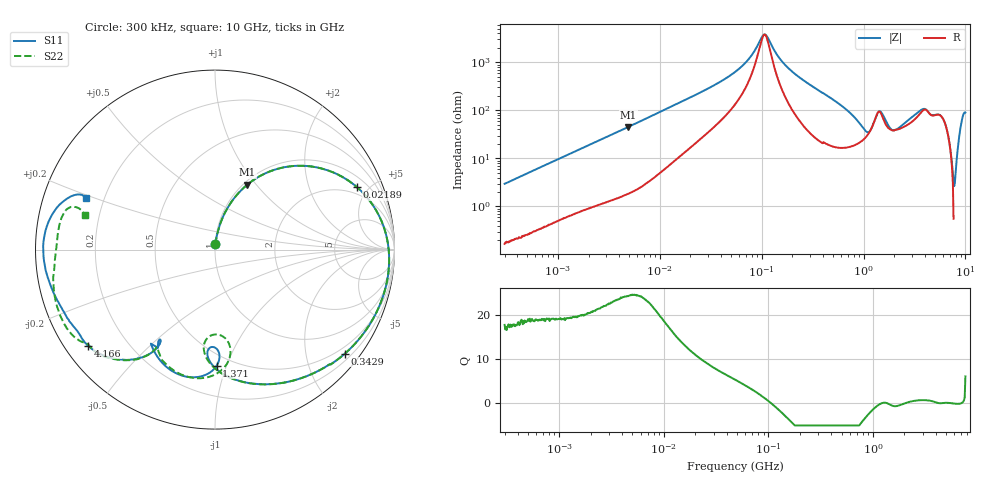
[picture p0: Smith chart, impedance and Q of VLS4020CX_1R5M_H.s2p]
! S-Parameter Data Generated by TDK Corporation
! Copyright(C) 2024 TDK Corporation.
! All Rights Reserved.
! TDK P/N: VLS4020CX-1R5M-H (SMD / SMT Inductor (Coil))
! Property: L=1.5uH at 1MHz
! Size(LxWxT): 4x4x2mm
! Model Type: s2p (Touchstone File Format Version 1.0)
! Frequency: DC=Yes Start=0.3MHz Stop=10000MHz 802points Log-sweep
! Model Generated on May 28, 2024
! Terms and conditions regarding TDK Simulation Models:
! 1)This simulation model is being provided solely for informational
!  purposes. Please refer to the specifications of the products in
!  terms of detailed characteristics of such products.
! 2)In no event shall TDK Corporation of any of its subsidiaries be
!  liable for any loss or damage arising, directly or indirectly,
!  from any information contained in this simulation model, including,
!  but not limited to loss or damages arising from any inaccuracies,
!  omissions or errors in connection with such information.
! 3)Any and all copyrights on this simulation model are owned by
!  TDK Corporation.  Duplication or redistribution of this simulation
!  model without prior written permission from TDK Corporation
!  is prohibited.
! 4)This simulation model is subject to any modification or change
!  without any prior notice.
! 5)Neither TDK Corporation nor any of its subsidiaries shall make any
!  warranty, express or implied, including but not limited to the
!  correctness, implied warranties of merchantability and fitness for
!  a particular purpose with respect to this simulation models.
! 6)The use of this simulation model shall be deemed to have consented
!  to the terms and conditions hereof.
! Port Assignments:
!  1 ---@@@--- 2
! Applicable Conditions:
!  Temperature = 25 degC
!  DC Bias Current = 0 A
!  Small Signal Operation
# Hz S MA R 50
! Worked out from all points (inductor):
!   801 points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, 300 kHz to 10 GHz, reference 50 ohm
!   read as one part in series: L = 1.56 uH near 318.3 kHz
!   highest Q = 24.6 at 4.921 MHz (marker M1), where L = 1.47 uH
!   self-resonance near 106.7 MHz
!   S11 on the Smith chart (normalised r, x): 300 kHz: 1.00, +0.06; 21.89 MHz: 1.54, +4.25; 342.9 MHz: 0.34, -2.81; 1.371 GHz: 0.42, -0.92; 4.166 GHz: 0.07, -0.33; 10 GHz: 0.13, +0.19
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300000  0.02934 85.0  0.998 -1.7  0.9978 -1.7  0.02926 85.1
1713600  0.1574 78.0  0.9796 -9.1  0.9796 -9.1  0.1573 78.0
4920797  0.4049 63.5  0.8981 -24.2  0.8979 -24.2  0.4049 63.5
9671944  0.6469 46.2  0.7295 -40.8  0.7295 -40.8  0.6468 46.2
2.189307e7  0.8649 23.6  0.425 -60.8  0.425 -60.8  0.8648 23.6
5.477226e7  0.9564 5.1  0.1528 -72.7  0.1527 -72.7  0.9564 5.1
1.080141e8  0.9744 -6.9  0.02557 -1.0  0.02558 -1.0  0.9743 -6.9
1.69821e8  0.9707 -16.7  0.1075 60.9  0.1075 60.9  0.9705 -16.7
3.126428e8  0.9368 -35.2  0.2708 49.6  0.2708 49.6  0.9367 -35.2
3.428535e8  0.927 -38.7  0.299 46.4  0.299 46.4  0.927 -38.7
5.82867e8  0.8337 -62.8  0.4659 21.4  0.4659 21.4  0.8327 -63.1
9.101824e8  0.6841 -87.5  0.5876 -11.0  0.5877 -11.0  0.6739 -88.9
1.196827e9  0.543 -92.0  0.5704 -44.2  0.5706 -44.2  0.4796 -92.8
1.371335e9  0.6467 -89.2  0.3982 -57.4  0.3983 -57.4  0.5867 -81.6
1.767019e9  0.6896 -116.2  0.4238 -52.6  0.4239 -52.6  0.7126 -108.5
2.629198e9  0.6063 -120.4  0.3639 -104.4  0.3637 -104.5  0.6527 -121.1
3.387826e9  0.7876 -128.7  0.1857 -134.9  0.185 -134.9  0.795 -129.1
4.166115e9  0.8881 -143.0  0.101 -126.6  0.101 -126.5  0.8759 -139.4
5.930102e9  0.9106 -157.6  0.0644 -131.6  0.06442 -131.6  0.9349 -152.0
7.652089e9  0.9568 -179.5  0.05247 -137.5  0.0523 -137.5  0.8941 -176.3
9.105558e9  0.8804 161.8  0.03934 -138.7  0.0393 -138.3  0.8639 165.9
1e10  0.775 158.1  0.03757 -130.9  0.03761 -130.7  0.747 165.0
